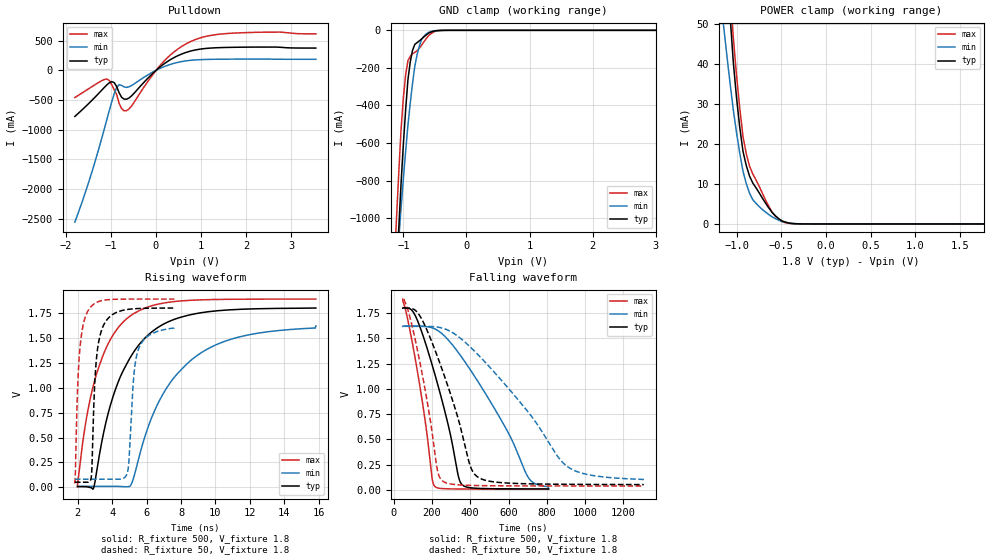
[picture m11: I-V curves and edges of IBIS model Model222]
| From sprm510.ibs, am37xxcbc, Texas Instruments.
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| Model based on original model for BQOMAPI2CHYFBPBRES_SSBHH
|   Sub model BQOMAPI2CHYRES_STD_PON_10_1P8
[model]   Model222
|[Input Load]   PU
|[Output Drive] LB10
|Voltage   1.8V
|Mode   I/O_OPEN_DRAIN
Model_type   I/O_open_drain
Polarity   Non-Inverting
Enable   Active-Low
Vinl =  0.567
Vinh =  1.323
Cref =  400.0000PF
Rref =  500.0000
Vref =  1.8V
Vmeas =  0.9
C_comp   3.85558p   3.723112p   3.857218p
[Model Spec]
Vinl   0.567   0.567   0.567
Vinh   1.323   1.323   1.323
[Temperature Range]   25   125   -40
[Voltage Range]   1.8   1.62   1.89
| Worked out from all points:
|   slope of the pulldown table from 0 to 0.27 V, typ, clamps not added: 1.71 ohm
|   GND clamp passes 1 mA (typ) near -0.44 V on its own axis
|   POWER clamp passes 1 mA (typ) near -0.51 V on its own axis
|   rising waveform, R_fixture 500, V_fixture 1.8: 20-80 % time 2.31ns typ, 3.14ns min, 1.76ns max; typ from 0.008 V to 1.8 V
|   rising waveform, R_fixture 50, V_fixture 1.8: 20-80 % time 345ps typ, 393ps min, 310ps max; typ from 0.052 V to 1.8 V
|   falling waveform, R_fixture 500, V_fixture 1.8: 20-80 % time 147ns typ, 293ns min, 92.6ns max; typ from 1.8 V to 0.008 V
|   falling waveform, R_fixture 50, V_fixture 1.8: 20-80 % time 174ns typ, 381ns min, 103ns max; typ from 1.8 V to 0.052 V
[POWER_clamp]
-1.8V     401.1mA    209.4mA    454.2mA
-1.145V   79.39mA    49.82mA    86.39mA
-1.073V   52.49mA    35.39mA    58.76mA
-1.036V   40.67mA    28.68mA    46.87mA
-963.6mV  24.19mA    17.73mA    28.97mA
-927.3mV  18.17mA    13.19mA    21.87mA
-890.9mV  14.63mA    10.1mA     17.61mA
-818.2mV  10.26mA    6.071mA    12.52mA
-600mV    2.834mA    1.747mA    2.888mA
-490.9mV  760.8uA    616.2uA    563.4uA
-381.8mV  112.8uA    147.2uA    57.34uA
1.764V    -11.66nA   -1.927uA   -18.08nA
[Pulldown]
-1.8V     -777.2mA   -2.558A    -458.6mA
-1.418V   -503.9mA   -1.705A    -274.5mA
-1.091V   -246.7mA   -833.5mA   -148.5mA
-927.3mV  -207.9mA   -396.6mA   -325.3mA
-818.2mV  -377.3mA   -241.3mA   -554.3mA
-709.1mV  -485.1mA   -279.3mA   -680.7mA
-600mV    -467.4mA   -278.5mA   -652.4mA
218.2mV   129.7mA    72.88mA    185.7mA
545.5mV   266.3mA    143.3mA    389.7mA
927.3mV   350mA      177.3mA    532.8mA
1.855V    388.5mA    188.2mA    630.6mA
3.545V    374.3mA    185.4mA    613.7mA
[GND_clamp]
-1.8V     -6.905A    -5.48A     -6.849A
-1.145V   -1.563A    -1.472A    -1.273A
-1.109V   -1.305A    -1.292A    -1.009A
-1.073V   -1.058A    -1.118A    -761.8mA
-1.036V   -819.4mA   -948.6mA   -530.3mA
-1V       -610.5mA   -793.2mA   -361.6mA
-927.3mV  -263.9mA   -507.2mA   -161.9mA
-890.9mV  -170.2mA   -389mA     -139.4mA
-818.2mV  -74.8mA    -191.7mA   -117.8mA
-745.5mV  -55.76mA   -81.74mA   -95.49mA
-600mV    -15.41mA   -10.81mA   -28.59mA
3.6V      0A         0A         0A
[Ramp]
dV/dt_f  1.0784867/0.14703388u  0.9675877/0.29242892u   1.13451/92.997788n
dV/dt_r 0.48439909/2.3670936n 0.31590512/3.2887875n 0.60377548/1.7777268n
R_load = 528.00
[Rising Waveform]
R_fixture = 500
V_fixture = 1.8
V_fixture_min = 1.62
V_fixture_max = 1.89
1.982ns   7.688mV    10.51mV    6.348mV
2.467ns   7.432mV    10.51mV    658.3mV
2.88ns    -17.79mV   10.51mV    1.008V
3.061ns   121.1mV    10.51mV    1.124V
3.868ns   808.4mV    10.52mV    1.476V
4.955ns   1.275V     7.148mV    1.709V
6.633ns   1.602V     832.5mV    1.838V
8.532ns   1.732V     1.269V     1.877V
11.11ns   1.785V     1.497V     1.888V
15.84ns   1.8V       1.62V      1.89V
[Rising Waveform]
R_fixture = 50
V_fixture = 1.8
V_fixture_min = 1.62
V_fixture_max = 1.89
1.826ns   51.8mV     82.19mV    37.94mV
2.088ns   51.8mV     82.19mV    1.328V
2.573ns   50.1mV     82.19mV    1.766V
2.804ns   138.8mV    82.19mV    1.82V
3.097ns   1.316V     82.19mV    1.857V
3.512ns   1.633V     82.19mV    1.879V
4.887ns   1.786V     151.5mV    1.89V
5.262ns   1.793V     1.133V     1.89V
5.584ns   1.796V     1.41V      1.89V
7.614ns   1.8V       1.62V      1.89V
[Falling Waveform]
R_fixture = 500
V_fixture = 1.8
V_fixture_min = 1.62
V_fixture_max = 1.89
47.93ns   1.8V       1.62V      1.89V
115.7ns   1.717V     1.622V     1.271V
161.7ns   1.482V     1.619V     728.7mV
201.3ns   1.238V     1.605V     113.2mV
212.7ns   1.163V     1.597V     39.19mV
338.8ns   130.1mV    1.358V     7.894mV
356.5ns   52.83mV    1.312V     7.618mV
581ns     9.599mV    627.4mV    6.537mV
705ns     8.588mV    116.8mV    6.425mV
809ns     7.688mV    10.51mV    6.348mV
[Falling Waveform]
R_fixture = 50
V_fixture = 1.8
V_fixture_min = 1.62
V_fixture_max = 1.89
56.03ns   1.8V       1.62V      1.89V
138.7ns   1.719V     1.62V      1.253V
188.5ns   1.519V     1.619V     729.9mV
227.3ns   1.33V      1.613V     210.4mV
255.1ns   1.184V     1.602V     88.43mV
335.8ns   714.9mV    1.521V     49.6mV
398.8ns   244.3mV    1.418V     43.8mV
447.4ns   117.4mV    1.326V     41.69mV
905.2ns   54.47mV    233.3mV    38.07mV
1.306us   51.8mV     82.19mV    37.94mV
